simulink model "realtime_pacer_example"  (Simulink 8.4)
settings: Solver=ode45  StartTime=0.0  StopTime=20  FixedStep=0.05  MaxStep=none  RelTol=1e-3
libraries: realtime_pacer_lib x2

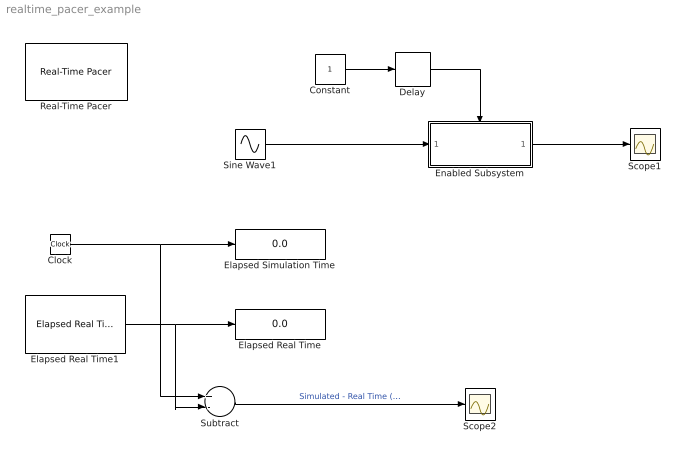
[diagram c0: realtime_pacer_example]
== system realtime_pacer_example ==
  Clock : Clock
  Constant : Constant
  Delay : Delay  DelayLength=5  InitialCondition=0
  Elapsed Real Time : Display
  Elapsed Real Time1 : realtime_pacer_lib/Elapsed Real Time
  Elapsed Simulation Time : Display
  Enabled Subsystem : Subsystem  TreatAsAtomicUnit=on
  Real-Time Pacer : realtime_pacer_lib/Real-Time Pacer  simTimePerRealTime=1
  Scope1 : Scope
  Scope2 : Scope
  Sine Wave1 : Sin  Frequency=2*pi*0.5  SampleTime=0
  Subtract : Sum  Inputs=+-
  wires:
  Clock/1 -> Elapsed Simulation Time/1, Subtract/1
  Sine Wave1/1 -> Enabled Subsystem/1(In1)
  Subtract/1 -> Scope2/1  "Simulated - Real Time (seconds)"
  Elapsed Real Time1/1 -> Elapsed Real Time/1, Subtract/2
  Enabled Subsystem/1(Out1) -> Scope1/1
  Constant/1 -> Delay/1
  Delay/1 -> Enabled Subsystem/Enable

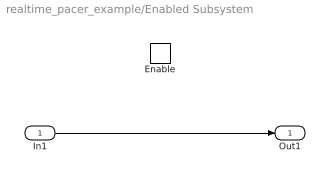
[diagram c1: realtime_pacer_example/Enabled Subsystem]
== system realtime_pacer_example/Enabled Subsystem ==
  In1 : Inport
  Enable : EnablePort
  Out1 : Outport
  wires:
  In1/1 -> Out1/1
